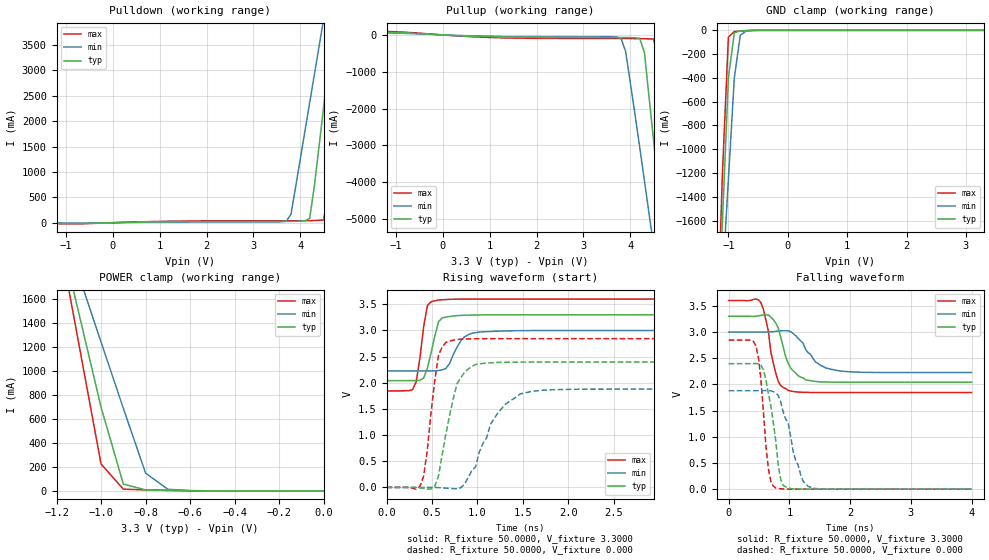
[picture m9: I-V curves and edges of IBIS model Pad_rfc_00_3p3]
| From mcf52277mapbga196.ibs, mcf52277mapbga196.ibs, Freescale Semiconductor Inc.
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|   Model Pad_rfc_00_3p3
[Model]   Pad_rfc_00_3p3
Model_type   3-state
Polarity   Non-Inverting
Enable   Active-High
Vmeas =   1.6500V
C_comp   1.7450pF   1.6200pF   1.8900pF
[Temperature Range]   25.0000   0.1500k   -40.0000
[Voltage Range]   3.3000V   3.0000V   3.6000V
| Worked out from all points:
|   slope of the pulldown table from 0 to 0.495 V, typ, clamps not added: 45 ohm
|   slope of the pullup table from 0 to 0.495 V, typ, clamps not added: 16.2 ohm
|   GND clamp passes 1 mA (typ) near -0.62 V on its own axis
|   POWER clamp passes 1 mA (typ) near -0.55 V on its own axis
|   rising waveform, R_fixture 50.0000, V_fixture 3.3000: 20-80 % time 103ps typ, 144ps min, 83.9ps max; typ from 2.04 V to 3.3 V
|   rising waveform, R_fixture 50.0000, V_fixture 0.000: 20-80 % time 169ps typ, 295ps min, 114ps max; typ from 0 V to 2.4 V
|   falling waveform, R_fixture 50.0000, V_fixture 3.3000: 20-80 % time 214ps typ, 318ps min, 171ps max; typ from 3.3 V to 2.04 V
|   falling waveform, R_fixture 50.0000, V_fixture 0.000: 20-80 % time 175ps typ, 271ps min, 124ps max; typ from 2.4 V to 0 V
[Pulldown]
| voltage   I(typ)   I(min)   I(max)
-3.3V     -260uA     -190uA     -310uA
-1V       -17.54mA   -7.821mA   -25.48mA
3.7V      26.67mA    29.81mA    37.67mA
3.8V      27.06mA    163.9mA    37.75mA
4.1V      35.36mA    1.809A     38.29mA
4.2V      83.91mA    2.362A     39.83mA
4.3V      724.2mA    2.915A     42.84mA
4.5V      2.292A     4.023A     53.33mA
4.7V      3.861A     5.131A     1.264A
4.9V      5.432A     6.24A      3.27A
5.1V      7.004A     7.35A      5.277A
6.6V      18.81A     15.69A     20.36A
[Pullup]
| voltage   I(typ)   I(min)   I(max)
-3.3V     111.1mA    97.6mA     129.3mA
-1.5V     87.16mA    67.14mA    107.7mA
1.2V      -56.36mA   -38.84mA   -76.64mA
3.8V      -71.64mA   -90.08mA   -99.03mA
3.9V      -72.46mA   -447.3mA   -99.27mA
4.2V      -92.61mA   -3.046A    -100.8mA
4.3V      -471.5mA   -3.954A    -103.1mA
4.5V      -2.906A    -5.767A    -111.2mA
4.7V      -5.407A    -7.59A     -1.297A
4.9V      -7.933A    -9.423A    -4.407A
5.1V      -10.46A    -11.26A    -7.529A
6.6V      -29.64A    -25.23A    -31.47A
[GND_clamp]
| voltage   I(typ)   I(min)   I(max)
-3.3V     -29.47A    -22.32A    -36.02A
-1.2V     -2.833A    -2.997A    -2.746A
-1.1V     -1.601A    -2.108A    -1.195A
-1V       -399mA     -1.252A    -56.61mA
-900mV    -20.31mA   -398.2mA   -10.19mA
-800mV    -5.193mA   -41.09mA   -5.939mA
-700mV    -2.389mA   -6.145mA   -2.797mA
-400mV    -10.19uA   -60.09uA   -3.537uA
3.3V      1.753nA    18.97uA    123.1pA
[POWER_clamp]
| voltage   I(typ)   I(min)   I(max)
-3.3V     18.78A     14A        23.32A
-1.2V     2.265A     2.345A     2.228A
-1.1V     1.481A     1.792A     1.226A
-1V       697mA      1.24A      224.1mA
-900mV    56.88mA    687.4mA    14.75mA
-800mV    8.425mA    147.7mA    8.532mA
-700mV    4.193mA    13.57mA    4.564mA
-500mV    349.8uA    802.1uA    248.4uA
0V        1.753nA    96.55nA    128.5pA
[Ramp]
| variable   typ   min   max
dV/dt_r   1.4375/0.1761n   1.1276/0.3107n   1.7066/0.1155n
dV/dt_f   0.7557/0.2179n   0.4637/0.3200n   1.0527/0.1661n
R_load = 50.0000
[Rising Waveform]
R_fixture = 50.0000
V_fixture = 3.3000
V_fixture_min = 3.0000
V_fixture_max = 3.6000
| time   V(typ)   V(min)   V(max)
0s        2.04V      2.227V     1.845V
285.7ps   2.043V     2.226V     1.869V
326.5ps   2.042V     2.227V     2.021V
408.2ps   2.092V     2.227V     3.071V
449ps     2.279V     2.228V     3.473V
530.6ps   2.889V     2.227V     3.567V
612.2ps   3.24V      2.247V     3.587V
857.1ps   3.291V     2.876V     3.599V
1.02ns    3.297V     2.969V     3.599V
4ns       3.3V       3V         3.6V
[Rising Waveform]
R_fixture = 50.0000
V_fixture = 0.000
| time   V(typ)   V(min)   V(max)
0s        1.228nV    337.4nV    -256.1pV
367.3ps   -5.839mV   93.21uV    18.8mV
408.2ps   -16.3mV    457.8uV    215.3mV
530.6ps   17.85mV    8.6uV      2.044V
653.1ps   1.025V     -12.89mV   2.772V
775.5ps   1.98V      -26.56mV   2.828V
857.1ps   2.198V     59.59mV    2.838V
1.143ns   2.382V     1.206V     2.843V
1.469ns   2.395V     1.788V     2.844V
4ns       2.396V     1.879V     2.844V
[Falling Waveform]
R_fixture = 50.0000
V_fixture = 3.3000
V_fixture_min = 3.0000
V_fixture_max = 3.6000
| time   V(typ)   V(min)   V(max)
0s        3.3V       3V         3.6V
530.6ps   3.319V     3V         3.559V
653.1ps   3.326V     2.999V     3.018V
693.9ps   3.285V     3.002V     2.62V
816.3ps   3.074V     3.02V      2.059V
979.6ps   2.402V     3.022V     1.885V
1.265ns   2.088V     2.674V     1.848V
1.429ns   2.056V     2.43V      1.846V
1.674ns   2.043V     2.291V     1.845V
4ns       2.04V      2.227V     1.845V
[Falling Waveform]
R_fixture = 50.0000
V_fixture = 0.000
| time   V(typ)   V(min)   V(max)
0s        2.396V     1.879V     2.844V
449ps     2.398V     1.879V     2.734V
530.6ps   2.367V     1.879V     2.092V
653.1ps   1.825V     1.883V     398.4mV
775.5ps   920.5mV    1.836V     23.33mV
816.3ps   452.7mV    1.789V     12.44mV
898ps     71.09mV    1.472V     4.629mV
1.102ns   5.479mV    554mV      577.7uV
1.306ns   1.327mV    57.3mV     83.59uV
4ns       2.828uV    42.21nV    2.832uV
